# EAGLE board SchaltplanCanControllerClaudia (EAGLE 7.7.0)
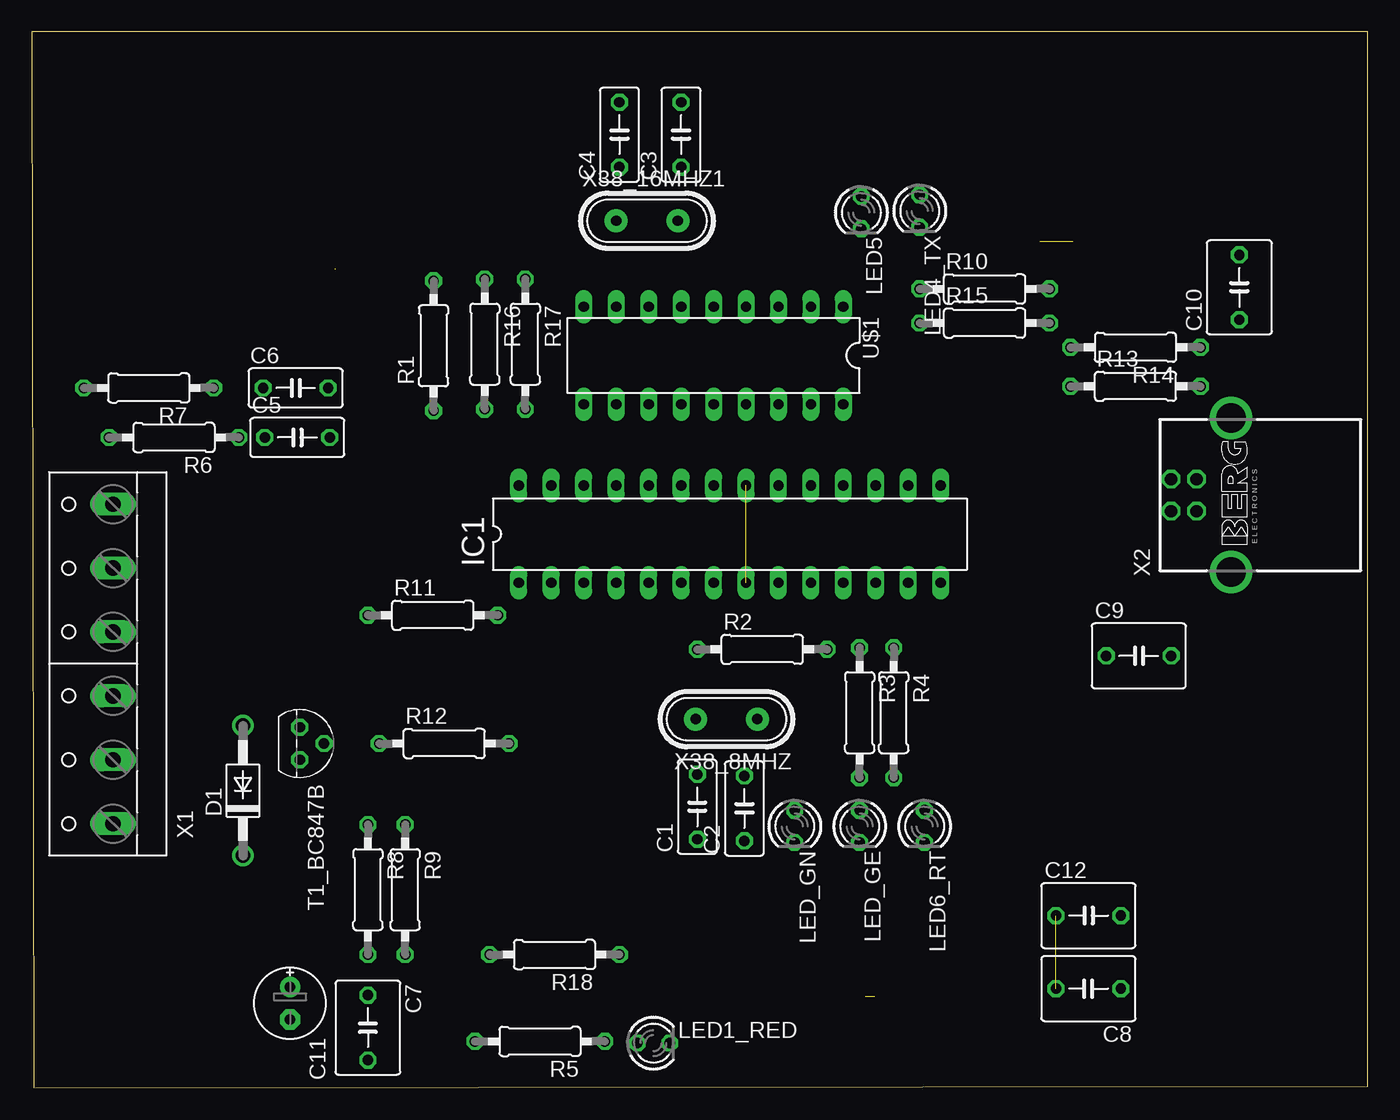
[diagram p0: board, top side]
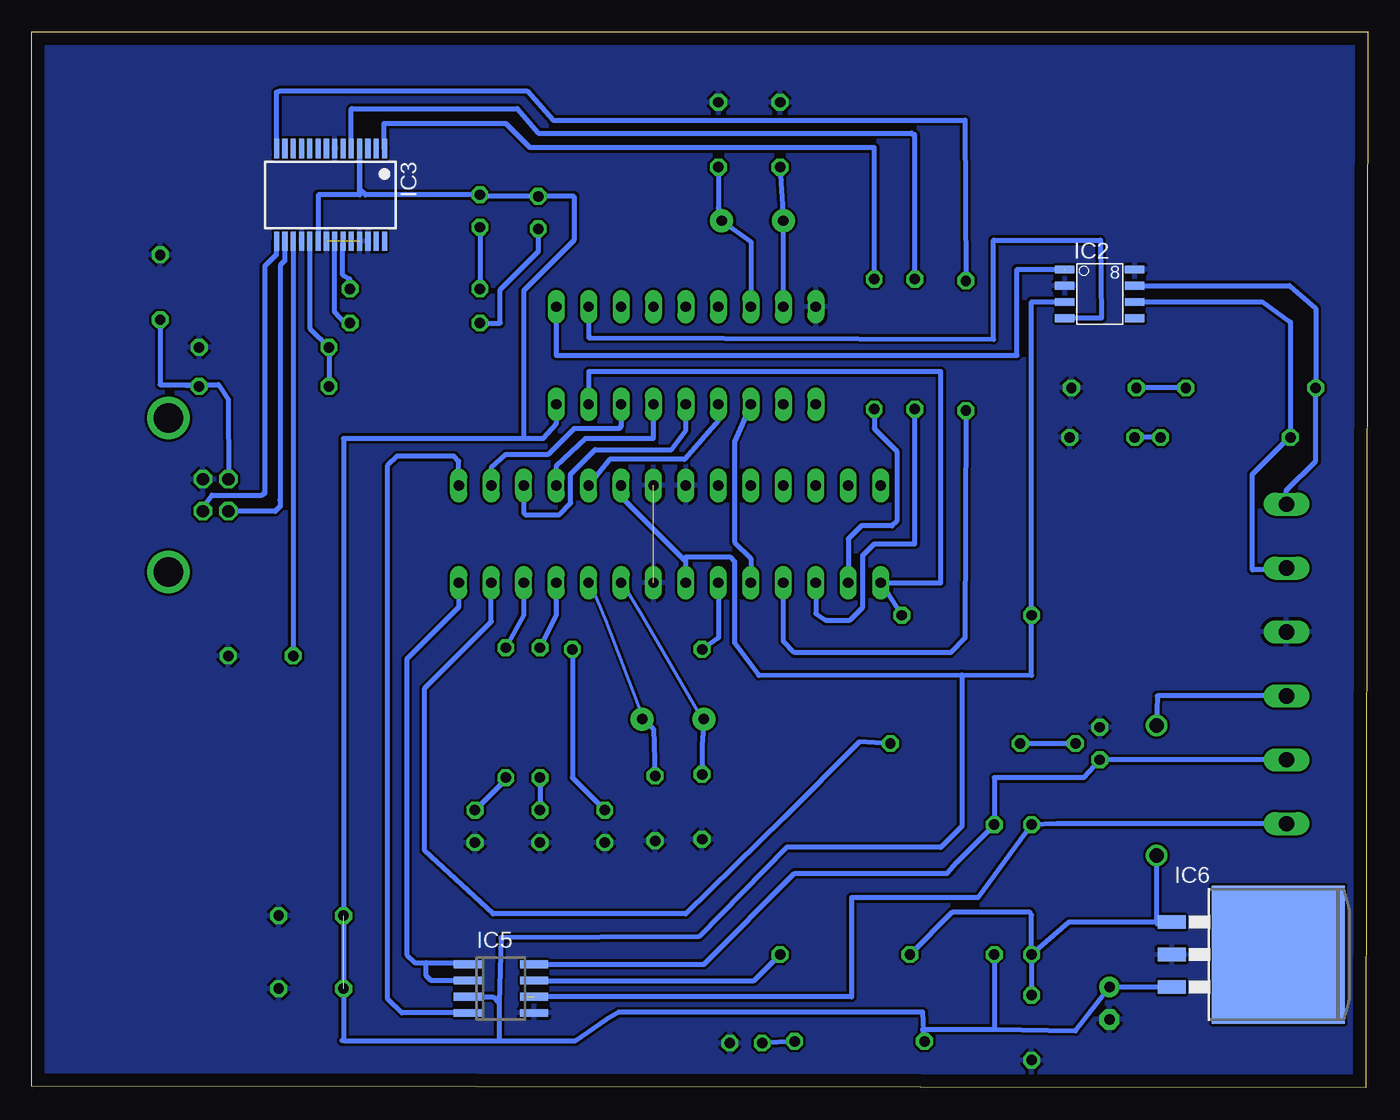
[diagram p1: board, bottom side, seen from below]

Size 104.52 x 82.59 mm. Coordinates in mm from the lower left corner, seen from the top.
Outline: 0.13,0 104.52,0.13 104.52,82.59 0,82.59 0.13,0
Copper layers (1*16): Top 0.035mm / dielectric 1.5mm / Bottom 0.035mm
Design rules "default": minimum track width 10mil, minimum drill 24mil, track to track 8mil, track to pad 8mil, pad to pad 8mil, via to via 8mil, smd to smd 8mil, copper to edge 40mil, drill to drill 8mil, minimum pad ring 10mil, minimum via ring 8mil, stop-mask expansion 4mil, vias tented up to drill 0mil, thermal gap 10mil

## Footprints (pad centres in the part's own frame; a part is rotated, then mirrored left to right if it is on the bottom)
C050-030X075 = drill 0.813 octagon: 1 -2.54,0; 2 2.54,0
C050-050X075 = drill 0.813 octagon: 1 -2.54,0; 2 2.54,0
E2,5-6E = drill 0.813 pad 1.575: + -1.27,0 | drill 0.813 pad 1.575 octagon: - 1.27,0
DO41-10 = drill 1.118: A 5.08,0; C -5.08,0
DIL28-3 = drill 0.813 long: 1 -16.51,-3.81; 2 -13.97,-3.81; 3 -11.43,-3.81; 4 -8.89,-3.81; 5 -6.35,-3.81; 6 -3.81,-3.81; 7 -1.27,-3.81; 8 1.27,-3.81; 9 3.81,-3.81; 10 6.35,-3.81; 11 8.89,-3.81; 12 11.43,-3.81; 13 13.97,-3.81; 14 16.51,-3.81; 15 16.51,3.81; 16 13.97,3.81; 17 11.43,3.81; 18 8.89,3.81; 19 6.35,3.81; 20 3.81,3.81; 21 1.27,3.81; 22 -1.27,3.81; 23 -3.81,3.81; 24 -6.35,3.81; 25 -8.89,3.81; 26 -11.43,3.81; 27 -13.97,3.81; 28 -16.51,3.81
DIL08 = smd 1.524 x 0.61: 1 -2.743,1.905; 2 -2.743,0.635; 3 -2.743,-0.635; 4 -2.743,-1.905; 5 2.743,-1.905; 6 2.743,-0.635; 7 2.743,0.635; 8 2.743,1.905
SSOP28 = smd 0.4 x 1.5: 1 -4.225,-3.625; 2 -3.575,-3.625; 3 -2.925,-3.625; 4 -2.275,-3.625; 5 -1.625,-3.625; 6 -0.975,-3.625; 7 -0.325,-3.625; 8 0.325,-3.625; 9 0.975,-3.625; 10 1.625,-3.625; 11 2.275,-3.625; 12 2.925,-3.625; 13 3.575,-3.625; 14 4.225,-3.625; 15 4.225,3.625; 16 3.575,3.625; 17 2.925,3.625; 18 2.275,3.625; 19 1.625,3.625; 20 0.975,3.625; 21 0.325,3.625; 22 -0.325,3.625; 23 -0.975,3.625; 24 -1.625,3.625; 25 -2.275,3.625; 26 -2.925,3.625; 27 -3.575,3.625; 28 -4.225,3.625
SO08 = smd 0.6 x 2.2: 1 -1.905,-2.6; 2 -0.635,-2.6; 3 0.635,-2.6; 4 1.905,-2.6; 5 1.905,2.6; 6 0.635,2.6; 7 -0.635,2.6; 8 -1.905,2.6
TO263-3 = smd 1.067 x 2.159: 1 -2.54,-5.791; 2 0,-5.791; 3 2.54,-5.791 | smd 10.8 x 10.41: TAB 0,2.54
LED3MM = drill 0.813 octagon: A -1.27,0; K 1.27,0
0207/10 = drill 0.813 octagon: 1 -5.08,0; 2 5.08,0
TO92 = drill 0.813 octagon: 1 1.27,0; 2 0,1.905; 3 -1.27,0
DIL18 = drill 0.813 long: 1 -10.16,-3.81; 2 -7.62,-3.81; 3 -5.08,-3.81; 4 -2.54,-3.81; 5 0,-3.81; 6 2.54,-3.81; 7 5.08,-3.81; 8 7.62,-3.81; 9 10.16,-3.81; 10 10.16,3.81; 11 7.62,3.81; 12 5.08,3.81; 13 2.54,3.81; 14 0,3.81; 15 -2.54,3.81; 16 -5.08,3.81; 17 -7.62,3.81; 18 -10.16,3.81
W237-6 = drill 1.194 long: 1 -12.5,-1.27; 2 -7.5,-1.27; 3 -2.5,-1.27; 4 2.5,-1.27; 5 7.5,-1.27; 6 12.5,-1.27
PN61729-S = drill 0.95 octagon: 1 1.25,4.71; 2 -1.25,4.71; 3 -1.25,2.71; 4 1.25,2.71 | drill 2.3 pad 2.9: S1 -6.02,0; S2 6.02,0
HC49 = drill 0.813 pad 1.8: 1 -2.413,0; 2 2.413,0

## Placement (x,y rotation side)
C1  22pF  [C050-030X075]  52.07,21.97 90 top
C2  22pF  [C050-030X075]  55.75,21.84 90 top
C3  22pF  [C050-030X075]  50.8,74.55 90 top
C4  22pF  [C050-030X075]  45.97,74.55 90 top
C5  560pF  [C050-030X075]  20.76,50.86 0 top
C6  560pF  [C050-030X075]  20.64,54.74 0 top
C7  100nF  [C050-050X075]  26.29,4.7 270 top
C8  100nF  [C050-050X075]  82.68,7.75 180 top
C9  100nF  [C050-050X075]  86.61,33.78 0 top
C10  10nF  [C050-050X075]  94.49,62.61 90 top
C11  10uf  [E2,5-6E]  20.19,6.6 270 top
C12  100nF  [C050-050X075]  82.68,13.46 0 top
D1  1N4004  [DO41-10]  16.51,23.24 90 top
IC1  MEGA48/88/168-PU  [DIL28-3]  54.61,43.31 0 top
IC2  SNOWND  [DIL08]  20.95,62.1 0 bottom
IC3  FT232RL  [SSOP28]  81.15,69.85 180 bottom
IC5  L9637D  [SO08]  67.82,7.75 270 bottom
IC6  LM2937  [TO263-3]  9.53,10.41 270 bottom
LED1_RED  2mA_+3,3V  [LED3MM]  48.64,3.49 0 top
LED4_TX  2mA_TX  [LED3MM]  69.47,68.58 270 top
LED5  2mA_RX  [LED3MM]  64.9,68.45 270 top
LED6_RT  2mA mC  [LED3MM]  69.85,20.45 270 top
LED_GE  2mA mC  [LED3MM]  64.77,20.45 270 top
LED_GN  2mA mC  [LED3MM]  59.69,20.45 270 top
R1  0  [0207/10]  31.43,58.04 90 top
R2  270  [0207/10]  57.15,34.29 0 top
R3  270  [0207/10]  64.77,29.34 270 top
R4  270  [0207/10]  67.44,29.34 270 top
R5  100  [0207/10]  39.75,3.62 180 top
R6  100  [0207/10]  11.11,50.86 180 top
R7  100  [0207/10]  9.14,54.74 180 top
R8  510  [0207/10]  26.29,15.49 270 top
R9  510  [0207/10]  29.21,15.49 270 top
R10  270  [0207/10]  74.55,62.48 0 top
R11  10k  [0207/10]  31.37,36.96 0 top
R12  1k  [0207/10]  32.26,26.92 0 top
R13  4k7  [0207/10]  86.36,54.86 0 top
R14  10k  [0207/10]  86.36,57.91 180 top
R15  270  [0207/10]  74.55,59.82 0 top
R16  0  [0207/10]  35.43,58.17 270 top
R17  0  [0207/10]  38.61,58.17 270 top
R18  0  [0207/10]  40.89,10.41 180 top
T1_BC847B  2N3565  [TO92]  20.95,26.92 270 top
U$1  MCP2515DIL  [DIL18]  53.34,57.28 180 top
X1  [W237-6]  5.08,33.15 90 top
X2  PN61729-S  [PN61729-S]  93.85,46.36 90 top
X38_8MHZ  CRYSTALS-NOGND-HC49  [HC49]  54.36,28.83 180 top
X38_16MHZ1  CRYSTALS-NOGND-HC49  [HC49]  48.13,67.82 0 top

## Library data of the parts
C1-C12 R1-R18 = rcl
D1 = diode
IC1 = avr-6
IC2 = SN65HVD231D
IC3 = ftdichip; MPN: FT232RL; OC_FARNELL: 1146032; OC_NEWARK: 91K9918
IC5 = st-microelectronics
IC6 = linear
LED1_RED LED4_TX LED5 LED6_RT LED_GE LED_GN = led
T1_BC847B = transistor
U$1 = MCP2515_MT
X1 = con-wago-500; OC_FARNELL: unknown; OC_NEWARK: unknown
X2 = con-berg; OC_FARNELL: unknown; OC_NEWARK: unknown
X38_8MHZ X38_16MHZ1 = IQD-Frequency-Products

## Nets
+5V: C8.2 C11.+ C12.1 IC1.7 IC1.20 IC2.3 IC3.4 IC3.20 IC5.3 IC6.3 LED4_TX.A LED5.A R5.2 R9.2 R11.1 U$1.18
+10V: C7.1 D1.C IC6.1 R8.2 R18.2
+12V: D1.A X1.3
GND: C1.1 C2.1 C3.2 C4.2 C5.2 C6.2 C7.2 C8.1 C9.2 C10.2 C11.- C12.2 IC1.8 IC1.21 IC1.22 IC2.2 IC2.8 IC3.7 IC3.18 IC3.21 IC3.25 IC3.26 IC5.5 IC6.2 LED1_RED.K LED6_RT.K LED_GE.K LED_GN.K R14.1 T1_BC847B.3 U$1.9 X1.4 X2.4
N$1: LED1_RED.A R5.1
N$2: IC1.1 R11.2 U$1.17
N$3: C1.2 IC1.9 X38_8MHZ.2
N$4: C5.1 R6.1
N$5: IC2.4 U$1.2
N$6: IC1.16 U$1.16
N$7: C2.2 IC1.10 X38_8MHZ.1
N$8: IC1.18 U$1.15
N$9: IC1.17 U$1.14
N$10: IC1.19 U$1.13
N$11: C3.1 U$1.7 X38_16MHZ1.2
N$12: C4.1 U$1.8 X38_16MHZ1.1
N$13: IC1.5 U$1.12
N$14: C6.1 R7.1
N$15: IC2.1 U$1.1
N$16: LED6_RT.A R4.2
N$17: IC1.14 IC5.1 IC5.2
N$18: IC1.15 IC5.4
N$19: IC3.16 X2.2
N$20: IC2.6 R6.2 X1.5
N$21: IC2.7 R7.2 X1.6
N$23: LED5.K R15.1
N$24: LED_GN.A R2.2
N$25: IC1.6 R2.1
N$26: IC1.11 R3.1
N$27: IC1.12 R4.1
N$28: LED_GE.A R3.2
N$29: IC3.15 X2.3
N$30: LED4_TX.K R10.1
N$31: IC1.2 R17.2
N$32: IC3.22 R15.2
N$33: IC5.6 R8.1 X1.1
N$34: R12.1 T1_BC847B.2
N$35: IC1.13 R12.2
N$36: IC5.8 R9.1 T1_BC847B.1 X1.2
N$37: C10.1 R13.2 X2.1
N$38: C9.1 IC3.17
N$39: IC3.23 R10.2
N$40: IC3.14 R1.2
N$41: IC1.4 R1.1
N$42: IC3.1 R17.1
N$43: IC5.7 R18.1
N$45: IC1.3 R16.2
N$46: IC3.5 R16.1
N$47: IC3.19 R13.1 R14.2

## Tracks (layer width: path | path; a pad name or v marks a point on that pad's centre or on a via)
+5V  (1 unrouted)
  Bottom 0.254: 53.49,39.68 IC1.7
  Bottom 0.406: IC1.7 53.34,41.15 | 53.34,41.15 53.34,41.53 49.91,41.53 49.53,41.15 49.53,34.8 47.62,32.26 31.74,32.28 | 31.74,32.28 26.29,32.26 R11.1 26.29,61.47 IC2.3 | 31.74,32.28 31.75,32.28 31.75,20.45 33.4,18.8 45.47,18.8 52.32,11.81 67.82,11.75 | U$1.18 63.5,51.94 64.52,50.8 66.04,50.8 | 66.04,50.8 80.14,50.8 C8.2 80.14,3.68 | 80.14,3.68 80.26,3.68 | 80.14,3.68 68.07,3.68 | 68.07,3.68 61.98,3.68 59.56,5.33 58.61,5.91 34.8,5.91 R5.2 34.8,4.57 29.21,4.57 | 78.87,69.85 78.87,70.3 | 78.87,70.3 78.87,73.46 IC3.4 78.88,69.86 78.87,69.85 | 78.87,69.85 82.11,69.85 82.11,66.31 IC3.20 | 66.04,50.8 66.04,62.36 62.1,66.29 62.1,69.72 LED5.A 69.34,69.72 LED4_TX.A 78.42,69.85 78.87,70.3 | IC1.20 58.42,46.23 53.34,41.15 | IC5.3 68.45,7.11 67.94,6.6 | 67.94,6.6 67.94,3.81 68.07,3.68 | 29.21,4.57 22.86,4.44 C11.+ IC6.3 | R9.2 29.21,4.57 | 67.75,11.49 67.82,11.75 | 67.82,11.75 67.94,6.6
+10V
  Bottom 0.406: D1.C 16.51,12.83 15.44,12.83 IC6.1 23.37,12.95 R8.2 | R8.2 C7.1 | R8.2 26.29,13.53 26.42,13.72 32.51,13.72 R18.2
+12V
  Bottom 0.406: X1.3 16.47,30.65 D1.A
GND  (2 unrouted)
  Top 0.254: 6.4,35.56 X1.4
  pour Bottom: 0,82.68 104.14,82.68 104.14,81.41 104.14,0.13 0,0.13
N$1
  Bottom 0.406: R5.1 LED1_RED.A
N$2
  Bottom 0.406: R11.2 IC1.1 33.4,39.5 33.4,56.01 60.96,56.01 U$1.17
N$3
  Bottom 0.254: IC1.9 58.29,39.45 56.77,36.96 51.99,28.75 X38_8MHZ.2
  Bottom 0.406: X38_8MHZ.2 52.07,26.8 C1.2
N$4
  Bottom 0.406: R6.1 C5.1
N$5
  Bottom 0.406: U$1.2 60.96,58.67 60.83,58.67 29.27,58.55 29.27,66.29 20.89,66.29 20.83,60.2 IC2.4
N$6
  Bottom 0.406: 58.42,51.82 58.55,51.56 | 58.55,51.56 62.1,51.56 64.14,49.53 67.44,49.53 68.58,48.51 IC1.16 | U$1.16 58.42,51.94 58.55,51.56
N$7
  Bottom 0.254: IC1.10 60.81,39.45 59.54,36.45 56.67,28.88 X38_8MHZ.1
  Bottom 0.406: X38_8MHZ.1 56.64,28.83 55.88,28.07 C2.2
N$8
  Bottom 0.406: IC1.18 63.5,48.64 61.21,50.8 55.88,50.8 U$1.15
N$9
  Bottom 0.406: IC1.17 66.04,44.96 65.91,44.83 63.25,44.83 62.36,45.72 62.36,48.01 60.45,49.91 54.48,49.91 53.34,51.44 U$1.14
N$10
  Bottom 0.406: U$1.13 50.8,52.2 53.47,49.15 59.31,49.15 IC1.19
N$11
  Bottom 0.406: C3.1 50.8,68.83 X38_16MHZ1.2 48.26,66.17 U$1.7
N$12
  Bottom 0.406: C4.1 X38_16MHZ1.1 U$1.8
N$13
  Bottom 0.406: U$1.12 49.53,50.55 49.53,42.67 48.26,41.4 IC1.5
N$14
  Bottom 0.406: R7.1 C6.1
N$15  (1 unrouted)
  Bottom 0.406: U$1.1 63.5,57.28 27.43,57.28 27.43,64.01 23.75,64.01
N$16
  Bottom 0.406: R4.2 67.31,24.26 LED6_RT.A
N$17
  Bottom 0.406: IC1.14 71.12,37.59 75.18,33.53 75.18,10.41 74.55,9.78 73.66,9.78 | 73.66,9.78 70.55,9.78 IC5.1 | 73.66,9.78 73.66,8.76 73.28,8.38 IC5.2
N$18
  Bottom 0.406: IC1.15 71.12,49.02 71.5,49.4 75.95,49.4 76.71,48.64 76.71,6.98 75.56,5.84 IC5.4
N$19
  Bottom 0.406: 85.11,45.96 85.09,45.47 | 85.09,45.47 85.47,45.09 89.12,45.09 X2.2 | IC3.16 84.73,64.69 85.09,64.32 85.09,45.47
N$20
  Bottom 0.406: IC2.6 8.26,61.47 6.03,59.88 R6.2 6.6,50.42 9.02,48.01 9.02,40.51 6.35,40.51 X1.5
N$21
  Bottom 0.406: IC2.7 6.1,62.74 4.06,60.96 R7.2 4.06,49.02 6.35,46.74 X1.6
N$23
  Bottom 0.406: LED5.K 64.9,65.41 67.88,62.42 67.88,59.82 R15.1
N$24
  Bottom 0.406: R2.2 62.23,24.26 LED_GN.A
N$25
  Bottom 0.406: IC1.6 50.8,35.18 R2.1
N$26
  Bottom 0.406: IC1.11 63.5,36.96 R3.1
N$27
  Bottom 0.406: IC1.12 66.04,36.96 R4.1
N$28
  Bottom 0.406: R3.2 LED_GE.A
N$29
  Bottom 0.406: X2.3 91.14,45.38 90.42,46.36 86.49,46.36 | 86.49,46.36 86.3,46.48 | IC3.15 85.41,66.13 85.41,65.15 86.3,64.26 86.3,46.55 86.49,46.36
N$30
  Bottom 0.406: LED4_TX.K R10.1
N$31
  Bottom 0.406: R17.2 38.61,51.56 36.83,49.78 36.83,44.32 37.21,43.94 39.62,43.94 40.64,42.93 IC1.2
N$32
  Bottom 0.406: R15.2 80.01,59.82 80.83,60.71 80.83,66.15 IC3.22
N$33  (1 unrouted)
  Bottom 0.406: X1.1 24.31,20.65 R8.1 30.48,14.86 40.39,14.86 40.39,7.11 65.91,7.11
N$34
  Bottom 0.406: T1_BC847B.2 R12.1
N$35
  Bottom 0.406: R12.2 39.75,27.05 45.72,21.08 53.34,13.59 68.45,13.59 73.79,18.54 73.79,31.24 68.58,36.45 IC1.13
N$36
  Bottom 0.406: IC5.8 51.94,9.65 44.83,16.76 32.89,16.76 32.13,17.65 R9.1 29.21,24.26 22.23,24.26 T1_BC847B.1 X1.2
N$37
  Bottom 0.406: R13.2 94.49,54.99 | 94.49,54.99 89.92,54.99 89.15,53.85 X2.1 | C10.1 94.49,54.99
N$38
  Bottom 0.406: IC3.17 84.08,36.07 C9.1
N$39
  Bottom 0.406: R10.2 79.63,63.25 80.2,63.56 80.2,65.99 IC3.23
N$40
  Bottom 0.406: IC3.14 85.38,77.88 85.09,77.98 65.79,77.98 63.75,75.69 31.5,75.69 R1.2
N$41
  Bottom 0.406: R1.1 31.5,35.18 32.64,34.04 44.83,34.04 45.72,34.93 IC1.4
N$42
  Bottom 0.406: R17.1 38.61,73.53 65.53,73.53 67.44,75.44 76.96,75.44 76.96,73.47 IC3.1
N$43
  Bottom 0.406: IC5.7 48.01,8.38 R18.1
N$45
  Bottom 0.406: IC1.3 43.18,37.08 42.42,36.58 40.51,36.58 39.5,37.59 39.5,41.66 38.61,42.55 35.43,42.55 R16.2
N$46
  Bottom 0.406: R16.1 35.43,74.42 | 35.43,74.42 35.43,74.55 | IC3.5 79.53,76.55 79.5,76.58 66.55,76.58 64.9,74.68 35.69,74.68 35.43,74.42
N$47
  Bottom 0.406: R13.1 R14.2 82.78,59.41 IC3.19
